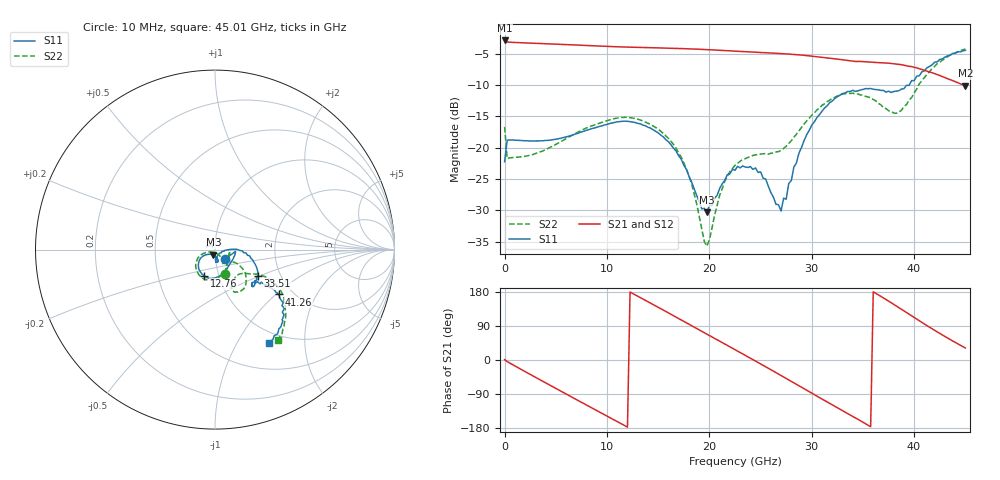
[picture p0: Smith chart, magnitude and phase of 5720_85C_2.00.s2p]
! Device:  ADRF5720
! Description: 0.5dB LSB GaAs MMIC 6-bit Digital Attenuator
! Frequency:  0.000009 -  40 GHz
! Ports:
!	RF1	= Port 1
!	RF2	= Port 2
! Vdd:  3.3 Volt
! Vss:  -3.3 Volt
! Control:  0/3.3 Volt
! State:  2.00 dB attenuation
! Data:  The device was measured using G-S-G Probes on a matrix board.
!  Data was collected using an calibrated 4 port network analyzer.
!  The reference plane for this measurement is at the launchers.
! Note:  Analog Devices supplies this data as a sample of measured data
!  for this product.  Your particular data for this product may vary.
!  Data was taken at 85 degrees C.
!  Analog Devices reserves the right to change this data at anytime.
# GHZ S DB R 45.0
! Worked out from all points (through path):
!   181 points, 10 MHz to 45.01 GHz, reference 45 ohm
!   highest |S21| = -2.86 dB at 10 MHz (marker M1); lowest = -10.1 dB at 45.01 GHz (marker M2)
!   group delay of S21, straight-line fit = 42.2 ps
!   lowest |S11| = -30.3 dB at 19.76 GHz (marker M3), VSWR 1.06, Z = 44.1 - j2.57 ohm
!   |S11| at or under -10 dB: start of sweep to 39.52 GHz
!   |S22| runs from -35.7 to -4.2 dB; largest |S21 - S12| = 0.0037
!   S11 on the Smith chart (normalised r, x): 10 MHz: 1.12, -0.12; 12.76 GHz: 0.85, -0.26; 33.51 GHz: 1.53, -0.49; 41.26 GHz: 1.70, -1.05; 45.01 GHz: 0.84, -1.37
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0.01  -22.23 -41.7  -2.86 1.0  -2.84 1.0  -16.68 -67.6
0.26  -18.80 -5.1  -3.11 -4.0  -3.10 -4.0  -21.72 -5.6
4.01  -18.84 -39.8  -3.38 -60.2  -3.36 -60.2  -20.31 -40.6
5.76  -18.37 -52.2  -3.50 -86.0  -3.48 -85.9  -18.79 -55.0
7.76  -17.37 -65.8  -3.65 -115.3  -3.63 -115.2  -17.04 -70.8
10.26  -16.14 -87.6  -3.82 -151.7  -3.80 -151.6  -15.55 -93.6
12.76  -15.97 -112.4  -3.96 172.1  -3.94 172.2  -15.35 -117.3
15.26  -17.99 -137.1  -4.06 135.4  -4.04 135.6  -17.38 -142.3
17.76  -23.45 -150.8  -4.19 98.3  -4.17 98.5  -23.36 -161.7
19.76  -30.32 -107.6  -4.33 68.4  -4.31 68.6  -35.74 -103.4
21.51  -25.22 -74.3  -4.47 42.2  -4.46 42.4  -25.36 -51.7
22.76  -22.98 -77.3  -4.59 23.5  -4.57 23.7  -22.50 -55.5
25.01  -23.87 -85.8  -4.79 -10.3  -4.77 -10.1  -21.02 -61.0
27.01  -30.11 -40.1  -4.96 -40.9  -4.94 -40.6  -20.40 -43.7
28.76  -20.85 1.3  -5.17 -68.0  -5.15 -67.7  -17.29 -32.8
30.26  -15.87 -6.2  -5.42 -91.4  -5.40 -91.2  -14.46 -34.9
33.51  -11.02 -31.9  -6.05 -141.5  -6.03 -141.2  -11.33 -55.5
35.76  -10.54 -43.9  -6.32 -176.2  -6.30 -175.8  -12.03 -67.0
37.76  -11.18 -41.4  -6.54 151.1  -6.52 151.5  -14.20 -55.7
38.76  -10.63 -38.8  -6.73 133.9  -6.71 134.3  -14.02 -42.0
41.26  -7.23 -35.0  -7.75 90.7  -7.73 91.0  -8.28 -29.7
45.01  -4.43 -59.9  -10.09 31.7  -10.06 32.1  -4.21 -55.0
